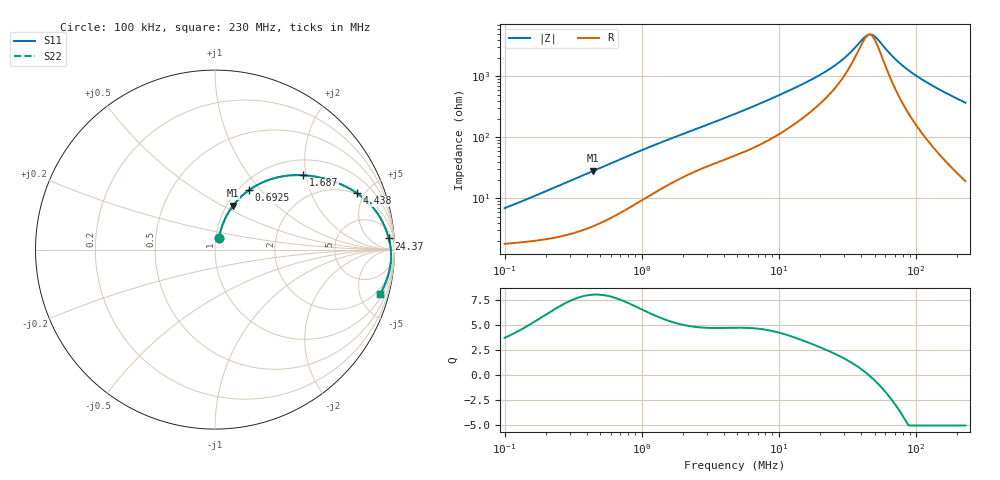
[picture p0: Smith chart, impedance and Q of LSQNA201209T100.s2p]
! LSQNA201209T100  S-PARAMETER MODEL  ( General Type )
! Model Generated by TAIYO YUDEN Corporation (http://www.ty-top.com)
! Version 2.0
! TAIYO YUDEN Control No. 100810NF25SB-FKC
! Copyright(c) 2007 TAIYO YUDEN CO.,LTD. All Rights Reserved.
! Product Description (link to TY-COMPAS)
! https://ds.yuden.co.jp/TYCOMPAS/or/detail?pn=LSQNA201209T100M&u=M
! Products Name : Inductors
! Characteristics :
!  Inductance : 10 uH , SRF(min) : 32 MHz , DC Resistance(max) : 1.3 Ohm
!  Rated Current : Saturation :205 mA , Temp Rise : 370 mA (40 degC)
!  Case Size : 2.0 x 1.25 / 0.079 x 0.049 [mm/inch] , Thickness : 0.9 / 0.035 [mm/inch]
!  (Conditions: Temperature = 25 degC , DC Bias Current/Voltage = 0A / 0V)
! External Node Assignments :
!  1  o---GGG---o  2
! GND o---------o GND
! Frequency Range : 0.1MHz  -  229.966873MHz  [ 402 STEP ]
# MHz S RI R 50
! Freq[MHz].  S11 Real  S11 Imag  S21 Real  S21 Imag  S12 Real  S12 Imag  S22 Real  S22 Imag
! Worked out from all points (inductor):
!   401 points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, 100 kHz to 230 MHz, reference 50 ohm
!   read as one part in series: L = 10.5 uH near 103.9 kHz
!   highest Q = 8.03 at 443.7 kHz (marker M1), where L = 10.1 uH
!   self-resonance near 45.55 MHz
!   S11 on the Smith chart (normalised r, x): 100 kHz: 1.04, +0.13; 692.5 kHz: 1.11, +0.86; 1.687 MHz: 1.37, +1.93; 4.438 MHz: 1.94, +4.42; 24.37 MHz: 12, +26; 230 MHz: 1.38, -7.40
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0.1  0.0218 0.0642  0.9782 -0.0642  0.9782 -0.0642  0.0218 0.0642
0.196855  0.0358 0.1201  0.9642 -0.1201  0.9642 -0.1201  0.0358 0.1201
0.365661  0.0761 0.209  0.9239 -0.209  0.9239 -0.209  0.0761 0.209
0.443732  0.1003 0.2446  0.8997 -0.2446  0.8997 -0.2446  0.1003 0.2446
0.692494  0.1894 0.3311  0.8106 -0.3311  0.8106 -0.3311  0.1894 0.3311
1.337081  0.4066 0.4123  0.5934 -0.4123  0.5934 -0.4123  0.4066 0.4123
1.686583  0.4928 0.4142  0.5072 -0.4142  0.5072 -0.4142  0.4928 0.4142
4.438293  0.7917 0.3138  0.2083 -0.3138  0.2083 -0.3138  0.7917 0.3138
4.889189  0.8137 0.2978  0.1863 -0.2978  0.1863 -0.2978  0.8137 0.2978
8.736987  0.9084 0.1971  0.0916 -0.1971  0.0916 -0.1971  0.9084 0.1971
17.53523  0.957 0.0979  0.043 -0.0979  0.043 -0.0979  0.957 0.0979
24.36589  0.968 0.0619  0.032 -0.0619  0.032 -0.0619  0.968 0.0619
30.73494  0.9736 0.0387  0.0264 -0.0387  0.0264 -0.0387  0.9736 0.0387
41.8889  0.9788 0.00837  0.0212 -0.00837  0.0212 -0.00837  0.9788 0.00837
45.26011  0.9797 0.000649  0.0203 -0.000649  0.0203 -0.000649  0.9797 0.000649
47.9654  0.9803 -0.00522  0.0197 0.00522  0.0197 0.00522  0.9803 -0.00522
50.83239  0.9807 -0.0112  0.0193 0.0112  0.0193 0.0112  0.9807 -0.0112
64.11956  0.9815 -0.0361  0.0185 0.0361  0.0185 0.0361  0.9815 -0.0361
80.87987  0.9801 -0.0636  0.0199 0.0636  0.0199 0.0636  0.9801 -0.0636
106.0471  0.975 -0.1002  0.025 0.1002  0.025 0.1002  0.975 -0.1002
153.1715  0.9593 -0.1605  0.0407 0.1605  0.0407 0.1605  0.9593 -0.1605
229.9669  0.9211 -0.245  0.0789 0.245  0.0789 0.245  0.9211 -0.245
